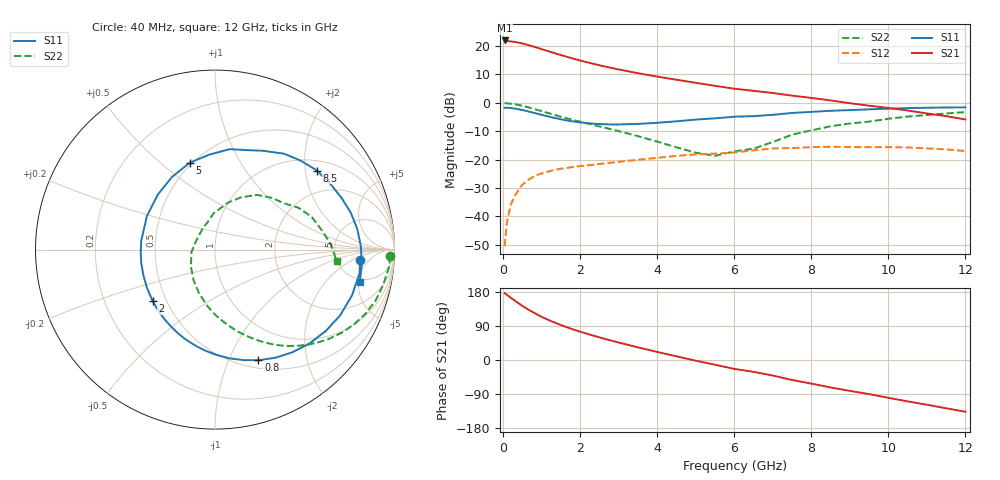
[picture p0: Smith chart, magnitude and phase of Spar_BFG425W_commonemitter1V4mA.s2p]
! Filename: 14bfg425.001
! BFG425W Field C1
! V1=8.281E-001V,V2=1.000E+000V, I1=5.607E-005A, I2=4.000E-003A
# GHz  S  MA  R 50
!  S11  S21  S12  S22
!Freq(GHz)  Mag  Ang  Mag  Ang  Mag  Ang  Mag  Ang
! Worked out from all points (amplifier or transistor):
!   44 points, 40 MHz to 12 GHz, reference 50 ohm
!   highest |S21| = 21.9 dB at 40 MHz (marker M1)
!   |S21| within 3 dB of that: start of sweep to 991.9 MHz
!   unconditionally stable (mu >= 1): 2.584 GHz to end of sweep
!   at 700 MHz: K = 0.29, MSG = 23.4 dB, |S12| = -26.7 dB
!   at 2.4 GHz: K = 0.94, MSG = 17.6 dB, |S12| = -21.7 dB
!   at 12 GHz: K = 1.54, MAG = 1.2 dB, |S12| = -17.0 dB
!   S11 on the Smith chart (normalised r, x): 40 MHz: 8.55, -2.95; 800 MHz: 0.59, -1.29; 2 GHz: 0.42, -0.30; 5 GHz: 0.49, +0.63; 8.5 GHz: 1.27, +2.32; 12 GHz: 4.49, -5.17
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0.04  0.811 -4.2  12.39 176.5  0.003 84.7  0.977 -2.2
0.1  0.816 -9.3  12.14 172.1  0.008 85.1  0.974 -5.8
0.2  0.805 -18.5  11.92 164.2  0.016 78.6  0.957 -11.9
0.3  0.788 -27.6  11.69 157.1  0.023 73.1  0.939 -17.6
0.4  0.766 -36.3  11.36 149.8  0.029 68.0  0.911 -23.2
0.5  0.742 -44.9  10.98 142.9  0.036 63.3  0.88 -28.2
0.6  0.716 -53.1  10.53 136.5  0.041 58.9  0.847 -32.9
0.8  0.662 -68.6  9.62 124.7  0.05 51.0  0.776 -41.6
1.1  0.586 -89.4  8.319 109.3  0.06 41.9  0.678 -52.4
1.4  0.527 -107.9  7.194 96.3  0.067 35.0  0.592 -61.3
1.7  0.481 -125.1  6.268 84.9  0.072 29.9  0.521 -68.9
2  0.45 -140.7  5.508 74.8  0.077 25.8  0.462 -75.8
2.2  0.435 -150.6  5.083 68.6  0.079 23.5  0.428 -80.2
2.6  0.418 -169.3  4.383 56.9  0.085 19.5  0.368 -89.0
3  0.414 173.4  3.833 46.1  0.091 15.6  0.316 -97.9
3.5  0.423 153.7  3.296 33.4  0.099 10.8  0.258 -110.4
4.5  0.47 120.8  2.527 9.7  0.116 0.1  0.164 -144.9
5  0.504 106.3  2.235 -1.9  0.123 -6.9  0.132 -174.0
6.5  0.579 73.3  1.611 -31.3  0.145 -21.4  0.155 106.5
8.5  0.719 37.7  1.095 -72.4  0.168 -55.1  0.384 52.5
10.5  0.801 8.2  0.728 -109.2  0.163 -88.2  0.569 18.6
12  0.827 -12.7  0.506 -136.5  0.141 -117.1  0.681 -5.4
